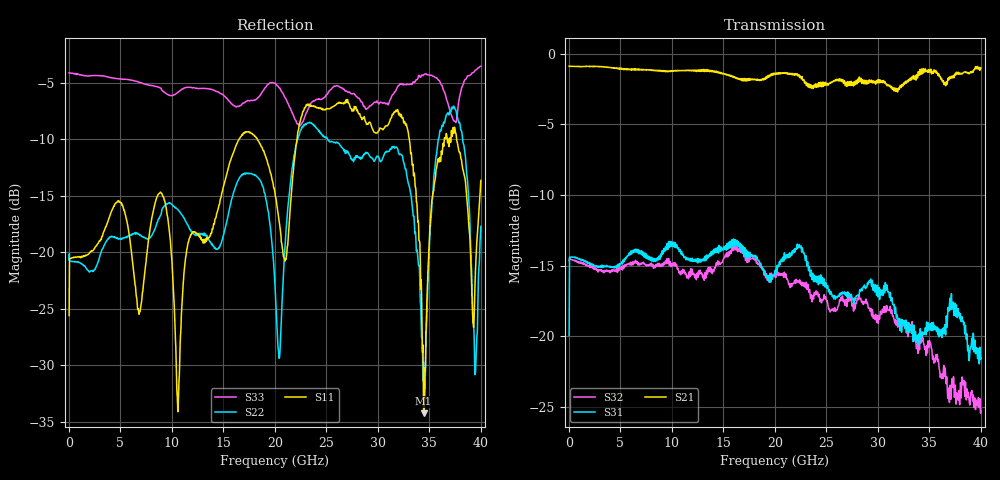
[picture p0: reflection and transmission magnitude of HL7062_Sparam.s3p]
! Created Wed Mar 30 16:27:32 2022
# ghz S ri R 50
! 3 Port Network Data from SP2.SP block
! freq  reS11  imS11  reS12  imS12  reS13  imS13
!  reS21  imS21
!  reS22  imS22  reS23  imS23
!  reS31  imS31  reS32  imS32
!  reS33  imS33
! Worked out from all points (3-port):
!   2000 points, 35 MHz to 40 GHz, reference 50 ohm
!   strongest paths, dB at 35 MHz, 10.03 GHz, 20.03 GHz, 30.02 GHz, 40 GHz:
!     S21: -0.9, -1.2, -1.4, -1.8, -1.0
!     S31: -19.9, -13.4, -15.4, -17.2, -21.5
!     S32: -14.6, -14.9, -15.5, -19.1, -25.3
!   lowest |S11| = -34.2 dB at 34.44 GHz (marker M1), VSWR 1.04, Z = 49.7 + j1.92 ohm
!   |S11| at or under -10 dB: start of sweep to 16.52 GHz; 18.3 GHz to 22.15 GHz (3.852 GHz wide, 19 % of centre); 33.06 GHz to 36.45 GHz (3.397 GHz wide, 9.77 % of centre)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
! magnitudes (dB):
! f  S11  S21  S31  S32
! 35 MHz  -25.6  -0.9  -19.9  -14.6
! 8.992 GHz  -14.8  -1.2  -14.4  -15.1
! 10.59 GHz  -34.1  -1.2  -13.8  -15.2
! 20.03 GHz  -14.8  -1.4  -15.4  -15.5
! 22.79 GHz  -7.5  -1.9  -14.1  -16.4
! 32.08 GHz  -7.7  -2.5  -18.8  -19.2
! 34.44 GHz  -34.2  -1.2  -19.9  -20.6
! 36.58 GHz  -9.9  -2.3  -19.9  -22.9
! 39.44 GHz  -22.5  -1.0  -20.5  -24.8
! 40 GHz  -13.6  -1.0  -21.5  -25.3
